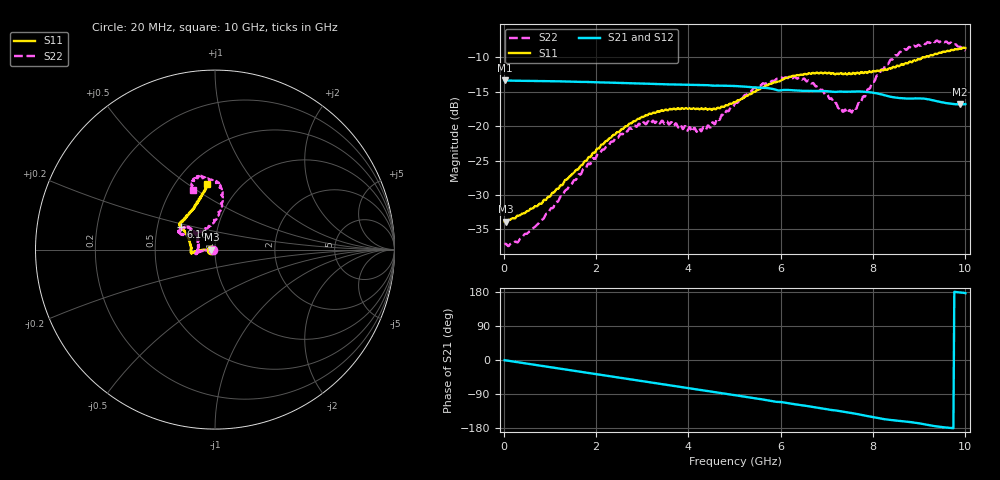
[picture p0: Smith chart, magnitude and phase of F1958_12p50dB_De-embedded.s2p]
! Integrated Device Technology
! Corporate Headquarters
! 6024 Silver Creek Valley Road
! San Jose, CA 95138  USA
! Phone:  1-408-284-8200
! Toll Free:  1-800-223-1366
! Webpage:  http://www.idt.com/
! Timing and RF Division
! 515 Groton Road, Suite 102
! Westford, MA 01886-6024
! Device:  F1958
! Description: 7-bit 0.25 dB Digital Step Attenuator
! Frequency:  0.001 -  6.000 GHz
! Package:  4x4 mm Thin QFN Plastic Package: 24 pin
! Ports:  2 RF, 12 DC
!  Pin  1  = D0
!  Pin  2  = VDD
!  Pin  3  = VMODE
!  Pin  4  = GND
!  Pin  5  = RF1  =  Port 1
!  Pin  6  = GND
!  Pin  7  = GND
!  Pin  8  = GND
!  Pin  9  = GND
!  Pin 10  = GND
!  Pin 11  = GND
!  Pin 12  = GND
!  Pin 13  = GND
!  Pin 14  = RF2  =  Port 2
!  Pin 15  = GND
!  Pin 16  = LE
!  Pin 17  = CLK
!  Pin 18  = DATA
!  Pin 19  = D6
!  Pin 20  = D5
!  Pin 21  = D4
!  Pin 22  = D3
!  Pin 23  = D2
!  Pin 24  = D1
! State:  50
! Atten State:  12.50 dB
! Voltage:  +3.30 Volts
! Current:  0.258 mA
! Data:  The device was measured on a F1958 evaluation board which has
!  individual transmission lines to the RF pins.  Data was collected
!  using a calibrated network analyzer.  The evaluation board was
!  de-embedded using Automatic Fixture Removal (AFR).
!  The reference plane is the edge of the package pin.
! Misc:
!  Action Tracker AT0419
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# GHz S dB R 50
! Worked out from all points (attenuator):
!   500 points, 20 MHz to 10 GHz, reference 50 ohm
!   highest |S21| = -13.33 dB at 20 MHz (marker M1); lowest = -16.8 dB at 9.88 GHz (marker M2)
!   lowest |S11| = -33.9 dB at 40 MHz (marker M3), VSWR 1.04, Z = 48 - j0.0936 ohm
!   |S11| at or under -10 dB: start of sweep to 9.069 GHz; 9.092691 GHz to 9.120103 GHz (27.41 MHz wide, 0.301 % of centre)
!   |S22| runs from -37.4 to -7.5 dB; largest |S21 - S12| = 0.00071
!   S11 on the Smith chart (normalised r, x): 20 MHz: 0.96, -0.00; 6.16 GHz: 0.66, +0.17; 10 GHz: 0.70, +0.60
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0.02  -33.84 -177.4  -13.33 -0.5  -13.33 -0.5  -37.21 -176.4
0.04  -33.88 -177.2  -13.34 -0.9  -13.34 -0.9  -37.08 -174.9
0.32  -32.98 179.3  -13.39 -6.1  -13.38 -6.1  -36.73 -178.5
0.72  -31.64 -178.9  -13.42 -13.6  -13.42 -13.6  -34.35 -175.2
1.7  -25.64 -177.9  -13.55 -31.7  -13.54 -31.7  -26.56 -175.7
2.6  -20.29 -175.5  -13.72 -48.3  -13.70 -48.3  -20.93 -172.8
2.92  -18.92 -173.3  -13.78 -54.2  -13.76 -54.3  -19.66 -170.0
3.36  -17.87 -171.6  -13.88 -62.3  -13.88 -62.4  -19.43 -166.2
4.3  -17.42 -178.4  -14.00 -79.4  -14.02 -79.5  -20.46 164.9
4.52  -17.56 175.6  -14.09 -83.6  -14.10 -83.7  -19.44 155.6
5.02  -16.49 161.7  -14.15 -92.9  -14.16 -92.9  -16.58 140.3
5.54  -14.64 151.0  -14.37 -102.8  -14.38 -102.8  -14.06 141.2
6.16  -12.89 146.7  -14.72 -113.9  -14.73 -113.9  -13.00 150.4
6.68  -12.29 143.9  -14.86 -123.4  -14.88 -123.3  -13.76 154.3
7.3  -12.26 137.5  -14.96 -135.3  -14.97 -135.1  -17.23 133.1
7.5  -12.31 134.7  -14.98 -139.2  -14.98 -139.1  -17.64 114.4
7.68  -12.28 131.7  -14.94 -143.1  -14.94 -143.0  -16.66 97.2
8.34  -11.59 116.0  -15.64 -157.8  -15.64 -157.9  -10.81 81.5
8.68  -10.94 109.1  -15.96 -162.1  -15.96 -162.0  -8.77 86.2
9.26  -9.64 101.1  -16.19 -173.1  -16.19 -173.1  -7.69 99.5
9.88  -8.69 97.2  -16.82 178.3  -16.85 178.3  -8.44 109.5
10  -8.62 96.9  -16.78 176.5  -16.81 176.6  -8.99 110.4
